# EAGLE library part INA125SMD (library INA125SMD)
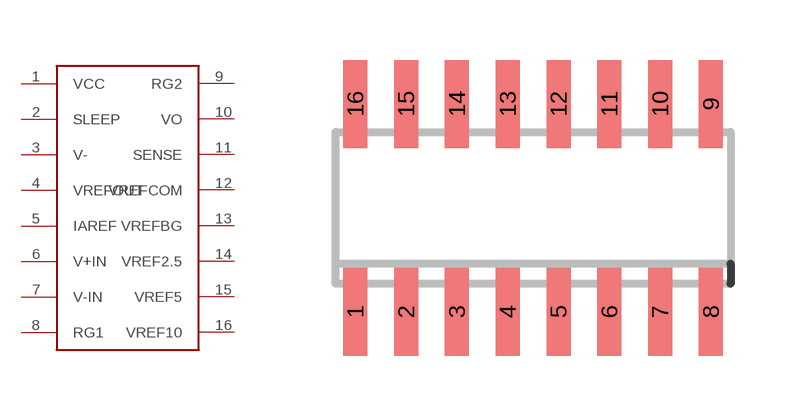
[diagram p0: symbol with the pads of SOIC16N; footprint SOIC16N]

Designator prefix -

## INA125SMD  [SOIC16N]
1  VCC
2  SLEEP
3  V-
4  VREFOUT
5  IAREF
6  V+IN
7  V-IN
8  RG1
9  RG2
10  VO
11  SENSE
12  VREFCOM
13  VREFBG
14  VREF2.5
15  VREF5
16  VREF10

## Footprint SOIC16N (pad centres in mm)
SMALL OUTLINE INTEGRATED CIRCUIT
smd 0.6 x 2.2: 1 -4.445,-2.6; 2 -3.175,-2.6; 3 -1.905,-2.6; 4 -0.635,-2.6; 5 0.635,-2.6; 6 1.905,-2.6; 7 3.175,-2.6; 8 4.445,-2.6; 9 4.445,2.6; 10 3.175,2.6; 11 1.905,2.6; 12 0.635,2.6; 13 -0.635,2.6; 14 -1.905,2.6; 15 -3.175,2.6; 16 -4.445,2.6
